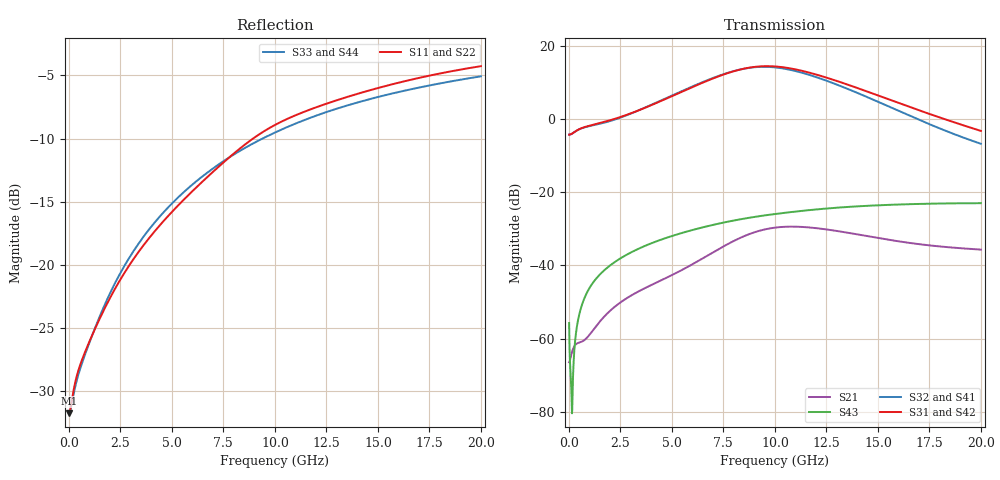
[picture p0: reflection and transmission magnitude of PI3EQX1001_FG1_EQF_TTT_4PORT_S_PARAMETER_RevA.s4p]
! NPort=4 DATA=2000 NOISE=0 GROUPDELAY=0 COMPLEX_DATAFORMAT=POLAR
! NumOfBlock=1 NumOfParam=0
! .MODEL Smodel S TSTONEFILE=PI3EQX1001_FG1_EQF_TTT_4PORT_S_PARAMETER_RevA.s4p TYPE=S
!  -- The above .MODEL line can be used for the S element in the netlist.
! The s parameter is extracted from the linear redriver, it is not bi-directional; only s(4,1)s(4,2) and s(3,1)s(3,2)
! should be the insertion loss
!Port definition:
!Port1 = input+
!Port2 = input¨C
!Port3 = output+
!Port4 = output-
# Hz S MA R  50
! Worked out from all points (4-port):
!   2000 points, 10 MHz to 20 GHz, reference 50 ohm
!   strongest paths, dB at 10 MHz, 5.01 GHz, 10.01 GHz, 15.01 GHz, 20 GHz:
!     S31: -4.3, 6.3, 14.4, 6.4, -3.3
!     S42: -4.3, 6.3, 14.4, 6.4, -3.3
!     S32: -4.3, 6.4, 14.1, 4.7, -6.8
!     S41: -4.3, 6.4, 14.1, 4.7, -6.8
!     S43: -55.8, -32.0, -26.0, -23.6, -23.0
!     S21: -66.5, -42.6, -29.7, -32.5, -35.7
!   lowest |S11| = -31.7 dB at 10 MHz (marker M1), VSWR 1.05, Z = 47.5 - j0.063 ohm
!   |S11| at or under -10 dB: start of sweep to 8.932 GHz
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1e7  0.02591 -178.5  0.0004939 2.7  3.669e-05 -0.2  4.787e-05 -0.1
     0.0004742 2.9  0.02597 -178.7  4.577e-05 -0.2  5.994e-05 -0.1
     0.612 -0.1  0.6119 179.9  0.02616 178.4  0.001614 -59.2
     0.6116 179.9  0.6117 -0.1  0.001627 -58.9  0.02612 178.4
6.66e9  0.2206 -105.4  0.01257 90.8  2.239e-05 -30.9  3.252e-05 -29.5
        0.01326 89.1  0.2189 -105.4  2.947e-05 -26.2  4.078e-05 -24.8
        3.283 -54.2  3.341 129.5  0.2301 -111.6  0.03398 57.7
        3.332 129.5  3.281 -54.1  0.03394 57.7  0.23 -111.6
8.64e9  0.3037 -107.1  0.02492 68.4  2.013e-05 -28.1  3.225e-05 -32.3
        0.02597 66.8  0.3018 -107.1  2.978e-05 -25.9  3.846e-05 -24.0
        4.968 -111.7  4.946 71.9  0.2935 -114.1  0.04421 45.4
        4.929 72.0  4.969 -111.6  0.04418 45.4  0.2932 -114.1
1.04e10  0.372 -112.0  0.03234 35.0  2.183e-05 -22.7  3.307e-05 -41.1
         0.03357 33.6  0.3693 -112.1  3.122e-05 -33.6  4.021e-05 -22.9
         5.096 -172.1  4.907 11.8  0.3459 -116.8  0.05206 34.2
         4.887 12.0  5.098 -171.9  0.05196 34.2  0.3456 -116.8
1.281e10  0.4434 -117.7  0.02902 -0.8  2.828e-05 -36.1  3.014e-05 -60.1
          0.0301 -2.0  0.4397 -117.8  2.854e-05 -50.8  4.593e-05 -33.2
          3.454 116.9  3.103 -58.1  0.4107 -120.8  0.06086 19.0
          3.088 -57.8  3.454 117.0  0.06075 19.1  0.4106 -120.7
1.543e10  0.5123 -122.6  0.02171 -19.6  2.813e-05 -67.8  2.255e-05 -87.5
          0.02259 -20.9  0.508 -122.6  2.07e-05 -74.4  4.312e-05 -55.2
          1.898 58.6  1.524 -113.0  0.4715 -124.9  0.067 2.9
          1.516 -112.6  1.898 58.7  0.06696 2.9  0.4712 -124.8
2e10  0.612 -130.6  0.01581 -27.0  1.401e-05 -151.2  1.141e-05 148.9
      0.01642 -29.1  0.6066 -130.6  6.981e-06 130.7  1.682e-05 -94.1
      0.6876 -13.8  0.4589 -167.2  0.5579 -131.2  0.07073 -23.2
      0.4577 -166.3  0.687 -13.7  0.07071 -23.2  0.5578 -131.1
